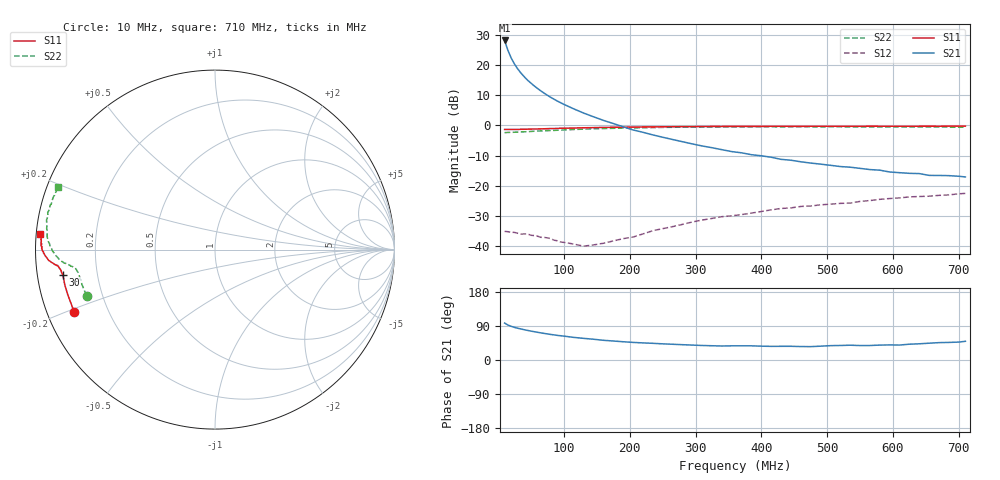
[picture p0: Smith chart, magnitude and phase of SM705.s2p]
!  POLYFET RF DEVICES
!  S PARAMETERS FOR
!  SM705
!  VDS=28, IDQ=600MA
! Date: Thu May 11 10:14:10 2000
# MHZ  S  MA  R  50.0000
! SCATTERING PARAMETERS :
! Freq=MHz Mag[s11] Ang[s11] Mag[s21] Ang[s21] Mag[s12] Ang[s12] Mag[s22] Ang[s22]
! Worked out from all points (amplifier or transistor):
!   60 points, 10 MHz to 710 MHz, reference 50 ohm
!   highest |S21| = 28.1 dB at 10 MHz (marker M1)
!   |S21| within 3 dB of that: start of sweep to 14.62 MHz
!   unconditionally stable (mu >= 1): 122.8 MHz to 246.7 MHz; 508.1 MHz to end of sweep
!   at 60 MHz: K = 0.36, MSG = 24.4 dB, |S12| = -36.6 dB
!   at 280 MHz: K = 0.94, MSG = 13.7 dB, |S12| = -32.7 dB
!   at 710 MHz: K = 1.15, MAG = 0.3 dB, |S12| = -22.5 dB
!   S11 on the Smith chart (normalised r, x): 10 MHz: 0.08, -0.21; 30 MHz: 0.08, -0.08; 710 MHz: 0.01, +0.04
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10  0.8581 -156.0  25.39 97.5  0.01779 8.0  0.7605 -160.2
15  0.8581 -163.2  17.47 92.3  0.01756 6.8  0.7672 -165.8
20  0.8597 -167.0  13.02 88.9  0.01716 5.0  0.7693 -168.7
25  0.8586 -169.2  10.35 86.0  0.01709 2.9  0.7726 -170.4
30  0.8597 -170.5  8.579 83.8  0.01654 2.0  0.7786 -171.4
35  0.8642 -171.5  7.306 81.8  0.01599 1.0  0.7812 -171.9
40  0.8653 -172.2  6.359 79.8  0.01615 0.2  0.7854 -172.5
45  0.8686 -172.7  5.583 78.0  0.01604 3.9  0.7901 -172.6
55  0.8749 -173.4  4.502 74.7  0.01515 0.4  0.8027 -173.3
65  0.879 -173.9  3.728 71.6  0.01418 1.3  0.8116 -173.7
75  0.8859 -174.2  3.155 68.8  0.01384 3.7  0.8199 -174.1
90  0.8927 -174.6  2.534 65.0  0.01243 8.3  0.8334 -174.7
115  0.9062 -175.2  1.881 59.7  0.01097 20.8  0.8582 -175.7
130  0.9157 -175.6  1.603 57.1  0.01012 31.8  0.8692 -176.4
160  0.9281 -176.3  1.214 52.0  0.0113 49.6  0.8895 -178.0
190  0.9364 -177.1  0.9515 48.2  0.01347 63.9  0.9069 -179.7
250  0.9503 -178.4  0.6392 42.6  0.01969 77.8  0.9297 177.2
310  0.9612 -179.6  0.4585 38.3  0.02737 84.2  0.9411 174.3
370  0.9661 179.4  0.3532 37.4  0.03365 86.1  0.9479 171.5
490  0.9708 177.6  0.2296 36.5  0.04883 87.8  0.9489 166.1
595  0.971 176.2  0.1702 39.8  0.06202 88.3  0.9477 162.2
710  0.9761 175.0  0.1409 49.4  0.07538 90.1  0.9406 158.2
